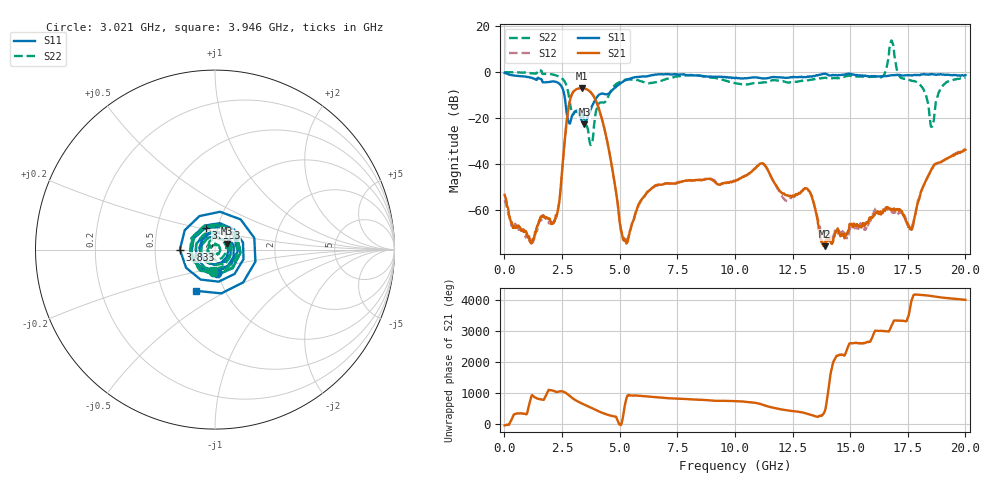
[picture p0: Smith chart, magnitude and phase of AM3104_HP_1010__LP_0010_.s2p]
!Created with skrf (http://scikit-rf.org).
# Hz S RI R 50.0
!freq ReS11 ImS11 ReS21 ImS21 ReS12 ImS12 ReS22 ImS22
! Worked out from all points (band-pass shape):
!   1601 points, 10 MHz to 20 GHz, reference 50 ohm
!   highest |S21| = -6.97 dB at 3.358 GHz (marker M1); lowest = -75.6 dB at 13.89 GHz (marker M2)
!   |S21| within 3 dB of the highest: 2.915 GHz to 3.841 GHz (925.1 MHz wide, 27.4 % of centre)
!   lowest |S11| = -22.6 dB at 3.471 GHz (marker M3), VSWR 1.16, Z = 57 + j3.75 ohm
!   |S11| at or under -10 dB: 2.601 GHz to 4.085 GHz (1.483 GHz wide, 44.4 % of centre)
!   |S22| runs from -31.7 to 13.7 dB; largest |S21 - S12| = 0.02
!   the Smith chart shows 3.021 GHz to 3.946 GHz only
!   S11 on the Smith chart (normalised r, x): 3.021 GHz: 0.99, -0.26; 3.183 GHz: 0.88, +0.22; 3.833 GHz: 0.67, +0.00; 3.946 GHz: 0.74, -0.36
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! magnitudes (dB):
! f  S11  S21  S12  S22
! 10 MHz  -0.4  -53.3  -55.6  -0.1
! 1.122 GHz  -2.3  -73.9  -73.5  -0.5
! 2.121 GHz  -4.1  -65.6  -65.2  -1.1
! 3.021 GHz  -17.6  -8.2  -8.2  -17.9
! 3.183 GHz  -17.6  -7.2  -7.3  -16.7
! 3.346 GHz  -20.9  -7.0  -7.1  -17.9
! 3.358 GHz  -21.2  -7.0  -7.0  -18.1
! 3.471 GHz  -22.6  -7.1  -7.2  -20.6
! 3.833 GHz  -14.2  -9.8  -9.9  -29.3
! 3.946 GHz  -12.0  -11.9  -11.9  -18.7
! 5.22 GHz  -3.7  -73.1  -73.2  -3.4
! 6.682 GHz  -1.0  -48.9  -49.1  -4.2
! 10.01 GHz  -2.7  -47.4  -47.2  -4.8
! 11.19 GHz  -2.8  -39.7  -39.9  -4.5
! 12.19 GHz  -2.5  -53.4  -55.7  -4.3
! 13.34 GHz  -2.0  -54.3  -53.8  -3.3
! 13.89 GHz  -0.7  -75.6  -69.9  -2.5
! 16.68 GHz  -1.5  -59.3  -60.1  7.2
! 17.65 GHz  -1.4  -68.2  -67.9  -3.8
! 18.54 GHz  -0.9  -41.9  -42.2  -23.7
! 19 GHz  -1.1  -38.7  -38.7  -6.2
! 20 GHz  -1.4  -33.7  -33.3  -2.5
